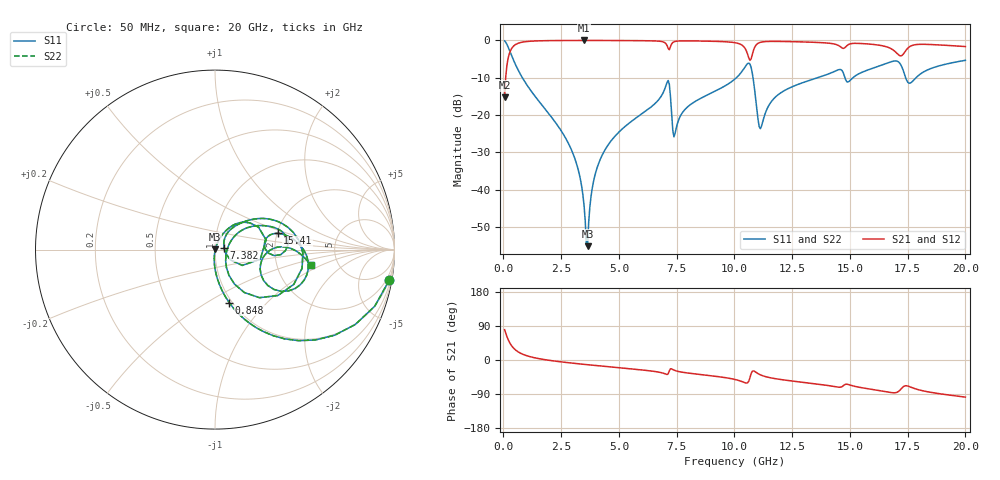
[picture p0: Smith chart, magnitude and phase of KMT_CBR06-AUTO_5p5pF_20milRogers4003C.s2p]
! Data measured by Modelithics Inc. support@modelithics.com 813-866-6335
! KEMET CBR06-AUTO 5.5pF, Pad Width= 0.851mm, Pad Length= 0.64mm, Pad Gap= 0.62mm, 20mil Rogers 4003C substrate Data, January 2022
# hz S ma R 50
! 2 Port Network Data from SP1.SP block
! freq  magS11  angS11  magS21  angS21  magS12  angS12  magS22  angS22
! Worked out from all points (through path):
!   401 points, 50 MHz to 20 GHz, reference 50 ohm
!   highest |S21| = -0.01 dB at 3.491 GHz (marker M1); lowest = -15.3 dB at 50 MHz (marker M2)
!   group delay of S21, straight-line fit = 15.3 ps
!   lowest |S11| = -55.2 dB at 3.641 GHz (marker M3), VSWR 1.00, Z = 50.2 + j0.0811 ohm
!   |S11| at or under -10 dB: 818.7 MHz to 10.09 GHz (9.266 GHz wide, 170 % of centre); 10.8 GHz to 13.6 GHz (2.8 GHz wide, 22.9 % of centre); 17.41 GHz to 17.86 GHz (448.8 MHz wide, 2.54 % of centre)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
!   |S22| runs from -55.2 to -0.1 dB; largest |S21 - S12| = 0
!   S11 on the Smith chart (normalised r, x): 50 MHz: 1, -11; 848 MHz: 0.97, -0.63; 7.382 GHz: 1.11, +0.02; 15.41 GHz: 2.01, +0.42; 20 GHz: 3.14, -0.78
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5e7  0.9851 -10.1  0.1716 79.9  0.1716 79.9  0.9851 -10.1
2.99375e8  0.6894 -47.4  0.7238 42.6  0.7238 42.6  0.6894 -47.4
8.48e8  0.3052 -75.0  0.9515 14.9  0.9515 14.9  0.3052 -75.0
2.74325e9  0.04578 -95.3  0.9977 -6.7  0.9977 -6.7  0.04578 -95.3
3.391625e9  0.01079 -94.1  0.9985 -10.9  0.9985 -10.9  0.01079 -94.1
3.491375e9  0.006041 -89.1  0.9986 -11.5  0.9986 -11.5  0.006041 -89.1
3.641e9  0.001742 27.7  0.9985 -12.4  0.9985 -12.4  0.001742 27.7
3.94025e9  0.01464 70.3  0.9984 -14.2  0.9984 -14.2  0.01464 70.3
4.389125e9  0.03376 70.6  0.9978 -16.8  0.9978 -16.8  0.03376 70.6
6.73325e9  0.1621 54.5  0.9769 -32.1  0.9769 -32.1  0.1621 54.5
7.13225e9  0.2898 10.7  0.7795 -36.3  0.7795 -36.3  0.2898 10.7
7.381625e9  0.05098 9.8  0.9583 -26.7  0.9583 -26.7  0.05098 9.8
1.0025e10  0.3043 34.7  0.9315 -51.3  0.9315 -51.3  0.3043 34.7
1.067338e10  0.4799 -23.8  0.5394 -46.4  0.5394 -46.4  0.4799 -23.8
1.112225e10  0.06554 -9.3  0.9422 -39.1  0.9422 -39.1  0.06554 -9.3
1.18205e10  0.1793 35.9  0.9699 -49.8  0.9699 -49.8  0.1793 35.9
1.336662e10  0.2993 26.5  0.9454 -61.9  0.9454 -61.9  0.2993 26.5
1.54115e10  0.3603 14.5  0.9109 -72.0  0.9109 -72.0  0.3603 14.5
1.670825e10  0.5078 -3.0  0.7948 -85.2  0.7948 -85.2  0.5078 -3.0
1.7207e10  0.4698 -29.4  0.6201 -76.8  0.6201 -76.8  0.4698 -29.4
1.7606e10  0.2671 -13.0  0.8314 -70.9  0.8314 -70.9  0.2671 -13.0
2e10  0.541 -9.4  0.8272 -98.0  0.8272 -98.0  0.541 -9.4
